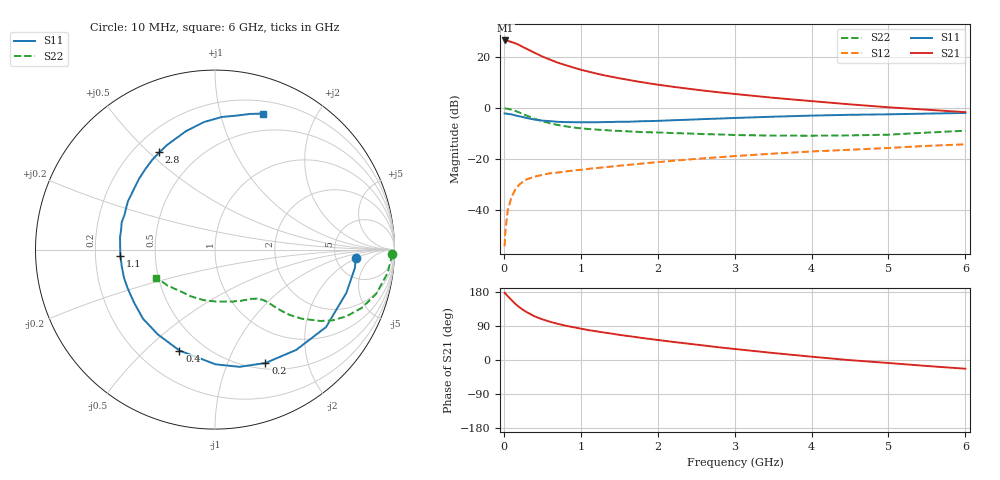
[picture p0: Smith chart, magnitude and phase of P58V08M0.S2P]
! SIEMENS Small Signal Semiconductors
! BFP183
! Si NPN RF Bipolar Junction Transistor in SOT143
! VCE = 8 V  IC = 8 mA
! Common Emitter S-Parameters:  March  1996
# GHz  S  MA  R  50
!  f  S11  S21  S12  S22
! GHz  MAG  ANG  MAG  ANG  MAG  ANG  MAG  ANG
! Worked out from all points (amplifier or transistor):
!   36 points, 10 MHz to 6 GHz, reference 50 ohm
!   highest |S21| = 26.4 dB at 20 MHz (marker M1)
!   |S21| within 3 dB of that: start of sweep to 277.8 MHz
!   unconditionally stable (mu >= 1): 1.385 GHz to 5.708 GHz
!   at 250 MHz: K = 0.26, MSG = 26.3 dB, |S12| = -28.7 dB
!   at 1.4 GHz: K = 1.01, MAG = 17.1 dB, |S12| = -22.9 dB
!   at 6 GHz: K = 0.96, MSG = 6.3 dB, |S12| = -14.2 dB
!   lowest NFmin = 1.30 dB at 450 MHz
!   S11 on the Smith chart (normalised r, x): 10 MHz: 7.83, -1.84; 200 MHz: 0.57, -1.38; 400 MHz: 0.37, -0.64; 1.1 GHz: 0.31, -0.03; 2.8 GHz: 0.30, +0.54; 6 GHz: 0.32, +1.36
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0.01  0.7843 -3.3  20.82 177.5  0.002 80.2  0.9863 -1.5
0.02  0.7863 -7.3  21 175.5  0.0039 81.7  0.9825 -3.2
0.05  0.7709 -18.1  20.69 168.5  0.0099 83.2  0.9699 -7.8
0.1  0.7544 -34.9  19.51 158.2  0.0182 72.2  0.9322 -15.2
0.15  0.719 -51.0  18.47 148.1  0.0258 65.1  0.8805 -21.6
0.2  0.6916 -66.0  17.11 139.6  0.0319 59.6  0.8213 -26.9
0.25  0.6673 -78.2  15.56 132.2  0.0367 54.6  0.7651 -31.0
0.3  0.639 -89.8  14.34 126.1  0.0407 50.9  0.7096 -34.1
0.4  0.5962 -109.4  12.08 115.2  0.0457 45.4  0.6187 -38.5
0.5  0.5699 -124.0  10.18 107.4  0.0494 41.5  0.5527 -41.2
0.6  0.5561 -136.1  8.877 101.0  0.0532 40.2  0.5052 -42.6
0.7  0.5396 -146.3  7.733 95.5  0.055 39.1  0.4685 -43.5
0.9  0.5308 -162.8  6.241 86.7  0.0601 38.1  0.4194 -44.8
1.1  0.528 -176.4  5.168 78.9  0.065 38.1  0.3902 -46.2
1.5  0.5416 163.7  3.837 66.4  0.0747 38.5  0.3576 -49.8
1.8  0.5547 151.0  3.201 58.1  0.0824 38.7  0.3398 -53.8
2.2  0.5788 137.0  2.612 47.8  0.0934 38.1  0.3245 -60.1
2.8  0.6243 119.8  2.031 33.4  0.1098 36.0  0.3053 -71.8
3.5  0.6789 103.9  1.592 18.5  0.1287 32.7  0.2899 -88.4
4.5  0.7398 87.1  1.184 -0.4  0.1535 26.4  0.2927 -117.0
5.5  0.7803 75.6  0.93 -15.8  0.1829 20.5  0.3318 -142.8
6  0.8036 70.6  0.833 -23.0  0.1959 16.4  0.3617 -154.5
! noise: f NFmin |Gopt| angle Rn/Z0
0.45  1.3  0.17  43  0.21
0.9  1.35  0.21  115  0.2
1.8  2.05  0.33  -177  0.14
